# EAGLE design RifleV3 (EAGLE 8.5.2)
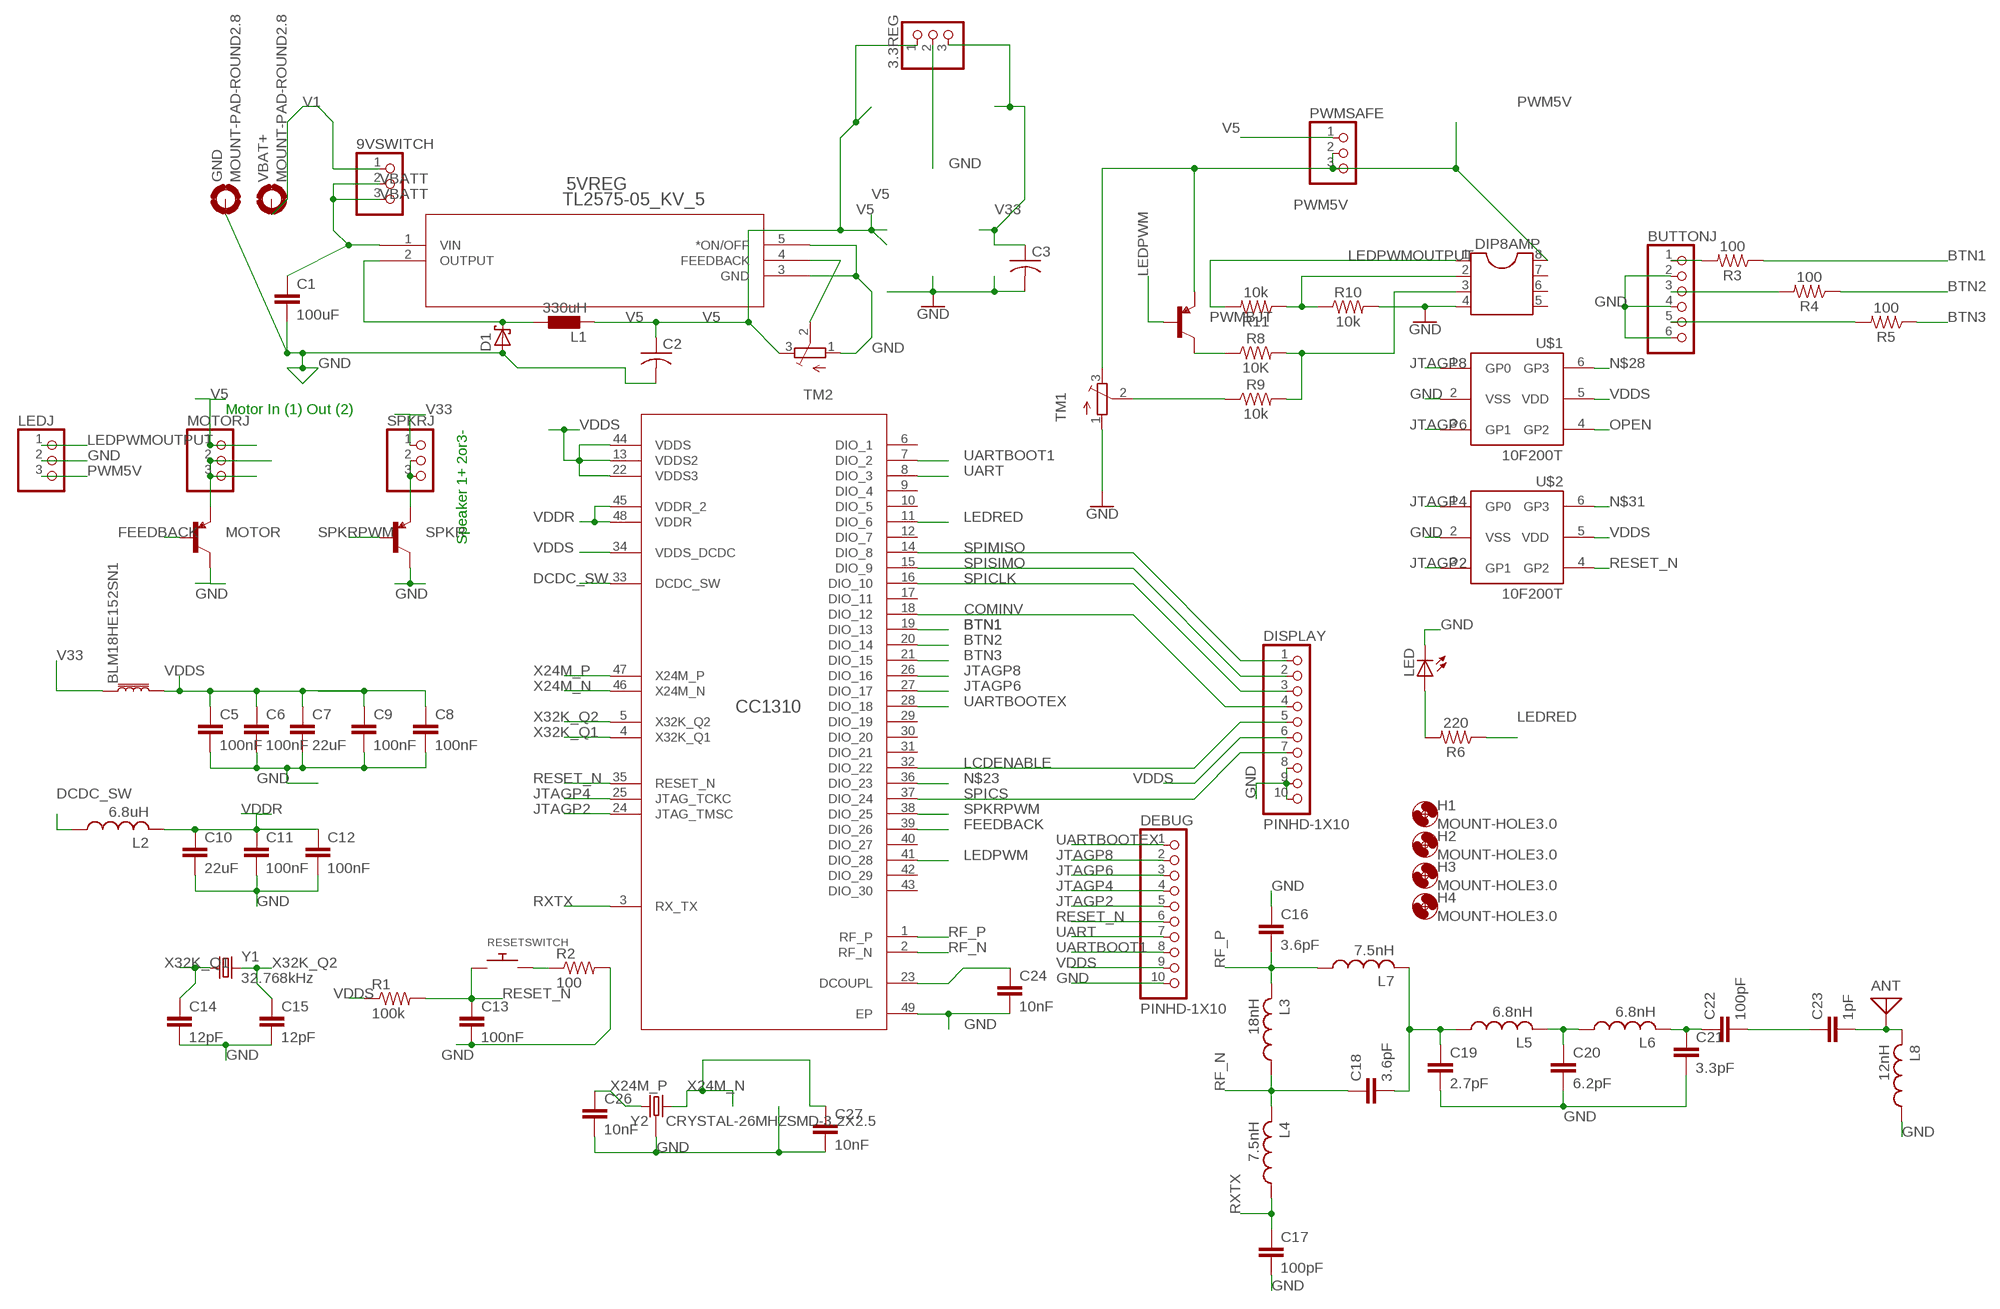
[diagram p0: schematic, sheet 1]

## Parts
3.3REG  PINHD-1X3CB  [1X03-CLEANBIG]
5VREG  TL2575-05_KV_5  [KV5]
9VSWITCH  PINHD-1X3  [1X03]
ANT  ANTENNA  [PAD-01]
BLM18HE152SN1  FERRITE_BEAD-0603  [0603]
BUTTONJ  PINHD-1X6  [1X06]
C1  100uF  10NF-PTH-10MM-10000V-1-%  [CAP-PTH-10MM]
C2  C-US025-024X044  [C025-024X044]
C3  C-US025-024X044  [C025-024X044]
C5  100nF  10NF-0603-50V-10%  [0603]
C6  100nF  10NF-0603-50V-10%  [0603]
C7  22uF  10NF-0603-50V-10%  [0603]
C8  100nF  10NF-0603-50V-10%  [0603]
C9  100nF  10NF-0603-50V-10%  [0603]
C10  22uF  10NF-0603-50V-10%  [0603]
C11  100nF  10NF-0603-50V-10%  [0603]
C12  100nF  10NF-0603-50V-10%  [0603]
C13  100nF  10NF-0603-50V-10%  [0603]
C14  12pF  10NF-0603-50V-10%  [0603]
C15  12pF  10NF-0603-50V-10%  [0603]
C16  3.6pF  10NF-0603-50V-10%  [0603]
C17  100pF  10NF-0603-50V-10%  [0603]
C18  3.6pF  10NF-0603-50V-10%  [0603]
C19  2.7pF  10NF-0603-50V-10%  [0603]
C20  6.2pF  10NF-0603-50V-10%  [0603]
C21  3.3pF  10NF-0603-50V-10%  [0603]
C22  100pF  10NF-0603-50V-10%  [0603]
C23  1pF  10NF-0603-50V-10%  [0603]
C24  10nF  10NF-0603-50V-10%  [0603]
C26  10nF  10NF-0603-50V-10%  [0603]
C27  10nF  10NF-0603-50V-10%  [0603]
CC1310  CC1310F128RGZR  [RGZ0048A]
D1  SCHOTTKY-DIODEDO41  [DO41-10]
DEBUG  PINHD-1X10  [1X10-BIG]
DIP8AMP  DIL8S  [SOCKET-08]
DISPLAY  PINHD-1X10  [1X10-BIG]
GND  MOUNT-PAD-ROUND2.8  [2,8-PAD]
H1  MOUNT-HOLE3.0  [3,0]
H2  MOUNT-HOLE3.0  [3,0]
H3  MOUNT-HOLE3.0  [3,0]
H4  MOUNT-HOLE3.0  [3,0]
L1  330uH  L0204/7  [0204/7]
L2  6.8uH  INDUCTOR_0603_M  [RESC0603_M]
L3  18nH  INDUCTOR_0603_M  [RESC0603_M]
L4  7.5nH  INDUCTOR_0603_M  [RESC0603_M]
L5  6.8nH  INDUCTOR_0603_M  [RESC0603_M]
L6  6.8nH  INDUCTOR_0603_M  [RESC0603_M]
L7  7.5nH  INDUCTOR_0603_M  [RESC0603_M]
L8  12nH  INDUCTOR_0603_M  [RESC0603_M]
LED  LEDCHIP-LED0805  [CHIP-LED0805]
LEDJ  PINHD-1X3  [1X03]
MOTOR  TRANSISTOR_PNPTO92  [TO-92]
MOTORJ  PINHD-1X3  [1X03]
PWMBJT  TRANSISTOR_PNPTO92  [TO-92]
PWMSAFE  PINHD-1X3  [1X03]
R1  100k  R-US_R0603  [R0603]
R2  100  R-US_R0603  [R0603]
R3  100  10MOHM-0603-1/10W-5%  [0603]
R4  100  10MOHM-0603-1/10W-5%  [0603]
R5  100  10MOHM-0603-1/10W-5%  [0603]
R6  220  10MOHM-0603-1/10W-5%  [0603]
R8  10K  10MOHM-0603-1/10W-5%  [0603]
R9  10k  10MOHM-0603-1/10W-5%  [0603]
R10  10k  10MOHM-0603-1/10W-5%  [0603]
R11  10k  10MOHM-0603-1/10W-5%  [0603]
RESETSWITCH  SWITCH_PUSHBUTTONSOFTTOUCHSMD_SJ  [PUSHBUTTON_SMD_SJ]
SPKR  TRANSISTOR_PNPTO92  [TO-92]
SPKRJ  PINHD-1X3  [1X03]
TM1  TRIMPOTTC33X  [TC33X]
TM2  TRIMPOTTC33X  [TC33X]
U$1  10F200T  [SOT23-6]
U$2  10F200T  [SOT23-6]
VBAT+  MOUNT-PAD-ROUND2.8  [2,8-PAD]
Y1  32.768kHz  FC-12M  [FC-12M]
Y2  CRYSTAL-26MHZSMD-3.2X2.5  [CRYSTAL-SMD-3.2X2.5MM]

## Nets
BTN1: CC1310.19(DIO_13) R3.1
BTN2: CC1310.20(DIO_14) R4.1
BTN3: CC1310.21(DIO_15) R5.1
COMINV: CC1310.18(DIO_12) DISPLAY.4
DCDC_SW: CC1310.33(DCDC_SW) L2.1
DCOUPL: C24.1 CC1310.23(DCOUPL)
FEEDBACK: CC1310.39(DIO_26) MOTOR.2(B)
GND: 3.3REG.2 5VREG.3(GND) 5VREG.5(*ON/OFF) BUTTONJ.2 BUTTONJ.4 BUTTONJ.6 C1.2 C2.2 C3.2 C5.2 C6.2 C7.2 C8.2 C9.2 C10.2 C11.2 C12.2 C13.2 C14.2 C15.2 C16.1 C17.2 C19.2 C20.2 C21.2 C24.2 C26.2 C27.2 CC1310.49(EP) D1.A DEBUG.10 DIP8AMP.4 DISPLAY.8 DISPLAY.9 DISPLAY.10 GND.B2,8(MOUNT) L8.1 LED.C LEDJ.2 MOTOR.3(C) R2.2 R10.2 SPKR.3(C) TM1.1(A) TM2.1(A) U$1.2(VSS) U$2.2(VSS) Y2.2 Y2.4
JTAGP2: CC1310.24(JTAG_TMSC) DEBUG.5 U$2.3(GP1)
JTAGP4: CC1310.25(JTAG_TCKC) DEBUG.4 U$2.1(GP0)
JTAGP6: CC1310.27(DIO_17) DEBUG.3 U$1.3(GP1)
JTAGP8: CC1310.26(DIO_16) DEBUG.2 U$1.1(GP0)
LCDENABLE: CC1310.32(DIO_22) DISPLAY.5
LEDPWM: CC1310.41(DIO_28) PWMBJT.2(B)
LEDPWMOUTPUT: DIP8AMP.1 LEDJ.1 R11.2
LEDRED: CC1310.11(DIO_6) R6.1
N$1: 5VREG.2(OUTPUT) D1.C L1.1
N$2: C22.2 C23.1
N$3: 5VREG.4(FEEDBACK) TM2.2(S)
N$4: MOTOR.1(E) MOTORJ.2 MOTORJ.3
N$5: C20.1 L5.2 L6.1
N$6: R2.1 RESETSWITCH.P$2
N$7: C18.2 C19.1 L5.1 L7.2
N$8: SPKR.1(E) SPKRJ.2 SPKRJ.3
N$9: ANT.1 C23.2 L8.2
N$10: R9.1 TM1.2(S)
N$11: PWMBJT.3(C) R8.1
N$12: BUTTONJ.1 R3.2
N$14: DIP8AMP.2 R10.1 R11.1
N$15: C21.1 C22.1 L6.2
N$16: DIP8AMP.3 R8.2 R9.2
N$17: BUTTONJ.3 R4.2
N$18: BUTTONJ.5 R5.2
N$22: LED.A R6.2
N$23: CC1310.36(DIO_23)
N$28: U$1.6(GP3)
N$31: U$2.6(GP3)
OPEN: U$1.4(GP2)
PWM5V: DIP8AMP.8 LEDJ.3 PWMBJT.1(E) PWMSAFE.2 PWMSAFE.3 TM1.3(E)
RESET_N: C13.1 CC1310.35(RESET_N) DEBUG.6 R1.2 RESETSWITCH.P$1 U$2.4(GP2)
RF_N: C18.1 CC1310.2(RF_N) L3.1 L4.2
RF_P: C16.2 CC1310.1(RF_P) L3.2 L7.1
RXTX: C17.1 CC1310.3(RX_TX) L4.1
SPICLK: CC1310.16(DIO_10) DISPLAY.3
SPICS: CC1310.37(DIO_24) DISPLAY.7
SPIMISO: CC1310.14(DIO_8) DISPLAY.1
SPISIMO: CC1310.15(DIO_9) DISPLAY.2
SPKRPWM: CC1310.38(DIO_25) SPKR.2(B)
UART: CC1310.8(DIO_3) DEBUG.7
UARTBOOT1: CC1310.7(DIO_2) DEBUG.8
UARTBOOTEX: CC1310.28(DIO_18) DEBUG.1
V1: 9VSWITCH.1 VBAT+.B2,8(MOUNT)
V5: 3.3REG.1 C2.1 L1.2 MOTORJ.1 PWMSAFE.1 TM2.3(E)
V33: 3.3REG.3 BLM18HE152SN1.1 C3.1 SPKRJ.1
VBATT: 5VREG.1(VIN) 9VSWITCH.2 9VSWITCH.3 C1.1
VDDR: C10.1 C11.1 C12.1 CC1310.45(VDDR_2) CC1310.48(VDDR) L2.2
VDDS: BLM18HE152SN1.2 C5.1 C6.1 C7.1 C8.1 C9.1 CC1310.13(VDDS2) CC1310.22(VDDS3) CC1310.34(VDDS_DCDC) CC1310.44(VDDS) DEBUG.9 DISPLAY.6 R1.1 U$1.5(VDD) U$2.5(VDD)
X24M_N: C27.1 CC1310.46(X24M_N) Y2.3
X24M_P: C26.1 CC1310.47(X24M_P) Y2.1
X32K_Q1: C14.1 CC1310.4(X32K_Q1) Y1.1
X32K_Q2: C15.1 CC1310.5(X32K_Q2) Y1.2
Unconnected: CC1310.6(DIO_1) CC1310.9(DIO_4) CC1310.10(DIO_5) CC1310.12(DIO_7) CC1310.17(DIO_11) CC1310.29(DIO_19) CC1310.30(DIO_20) CC1310.31(DIO_21) CC1310.40(DIO_27) CC1310.42(DIO_29) CC1310.43(DIO_30) DIP8AMP.5 DIP8AMP.6 DIP8AMP.7

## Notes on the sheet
- Motor In (1) Out (2)
- Speaker 1+ 2or3-

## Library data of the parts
3.3REG 9VSWITCH LEDJ MOTORJ PWMSAFE SPKRJ = adafruit:PINHD-1X3: PIN HEADER
5VREG = LM2575:TL2575-05_KV_5; DATASHEETURL: httpwww.ti.comlitgpnTL257505; FAMILY_NAME: STEPDOWN REGULATOR; GENERIC_PART_NUMBER: TL257505; INDUSTRY_STD_PKG_TYPE: TO220; MANUFACTURER: Texas Instruments; MANUFACTURER_PART_NUMBER: tl257505_kv_5; PACKAGE_DESIGNATOR: KV; PIN_COUNT: 5; VENDOR: Texas Instruments
ANT = discrete:ANTENNA: Antenna
BLM18HE152SN1 = SparkFun-Coils:FERRITE_BEAD: Ferrite Bead (blocks, cores, rings, chokes, etc.); PROD_ID: NDUC-07859; VALUE: 30Ω/1.8A
BUTTONJ = adafruit:PINHD-1X6: PIN HEADER
C1 = SparkFun-Capacitors:10NF: 0.01uF/10nF/10,000pF ceramic capacitors; PROD_ID: CAP-09321; VALUE: 10nF
C2 C3 = adafruit:C-US: CAPACITOR, American symbol
C5-C23 = SparkFun-Capacitors:10NF: 0.01uF/10nF/10,000pF ceramic capacitors; PROD_ID: CAP-00867; VALUE: 10nF
C24 C26 C27 = SparkFun-Capacitors:10NF: 0.01uF/10nF/10,000pF ceramic capacitors; PROD_ID: CAP-00867
CC1310 = CC1310RGZ:CC1310F128RGZR; ALTERNATEPARTNUMBER: CC1310F128RGZT; APPLICATION_BUILDNUMBER: *; COMPTYPE: IC; MANUFACTURER: Texas Instruments; MOUNTTYPE: SMT; PACKAGEREFERENCE: RGZ0048A; PARTNUMBER: CC1310F128RGZR; PIN_COUNT: 49; REFDES: RefDes; TYPE: TYPE; VALUE: Value
D1 = adafruit:SCHOTTKY-DIODE: Schottky Diode
DEBUG DISPLAY = adafruit:PINHD-1X10: Pin header 1x10 0.1" spacing With round pins
DIP8AMP = ic-package:DIL8: Dual In Line / Socket
GND VBAT+ = holes:MOUNT-PAD-ROUND: MOUNTING PAD, round
H1-H4 = holes:MOUNT-HOLE: MOUNTING HOLE with drill center marker
L1 = eagle-ltspice:L: INDUCTOR, European symbol; SPICEMODEL: NONE; SPICEPREFIX: L
L2-L8 = Nordic_nRF:INDUCTOR: Generic chip inductor
LED = adafruit:LED: LED
MOTOR PWMBJT SPKR = User-Submitted:TRANSISTOR_PNP: Generic PNP BJT Double check pinouts against datasheets- not all devices are the same! MMBT3906 - 40V 200mA SOT-23 (TRANS-08052) MMBT4403 - 40V 600mA SOT-23 (TRANS-09245)
R1 R2 = adafruit:R-US_: RESISTOR, American symbol
R3-R6 R8-R11 = SparkFun-Resistors:10MOHM: RES-09327; PROD_ID: RES-08283; VALUE: 10M
RESETSWITCH = adafruit:SWITCH_PUSHBUTTON: Buttons
TM1 TM2 = adafruit:TRIMPOT: SMT trimmer potentiometer part number TC33X http://www.ladyada.net/library/eagle
U$1 U$2 = adafruit:10F200T: PIC10F200/202/204/206 Ultra-small 8-bit PIC micros in SOT-23-6 and SOIC
Y1 = crystal:FC-12M: kHz RANGE CRYSTAL UNIT
Y2 = SparkFun-Clocks:CRYSTAL-26MHZ: 26MHz Crystal w/ Ground Pin Digikey Example Frequency: 26MHz Frequency Stability: &plusmn;9ppm Frequency Tolerance: &plusmn;10ppm Load Capacitance: 9pF SparkFun Products: SparkFun ESP32 Thing SparkFun ESP8266 Thing Dev Board; PROD_ID: XTAL-12454

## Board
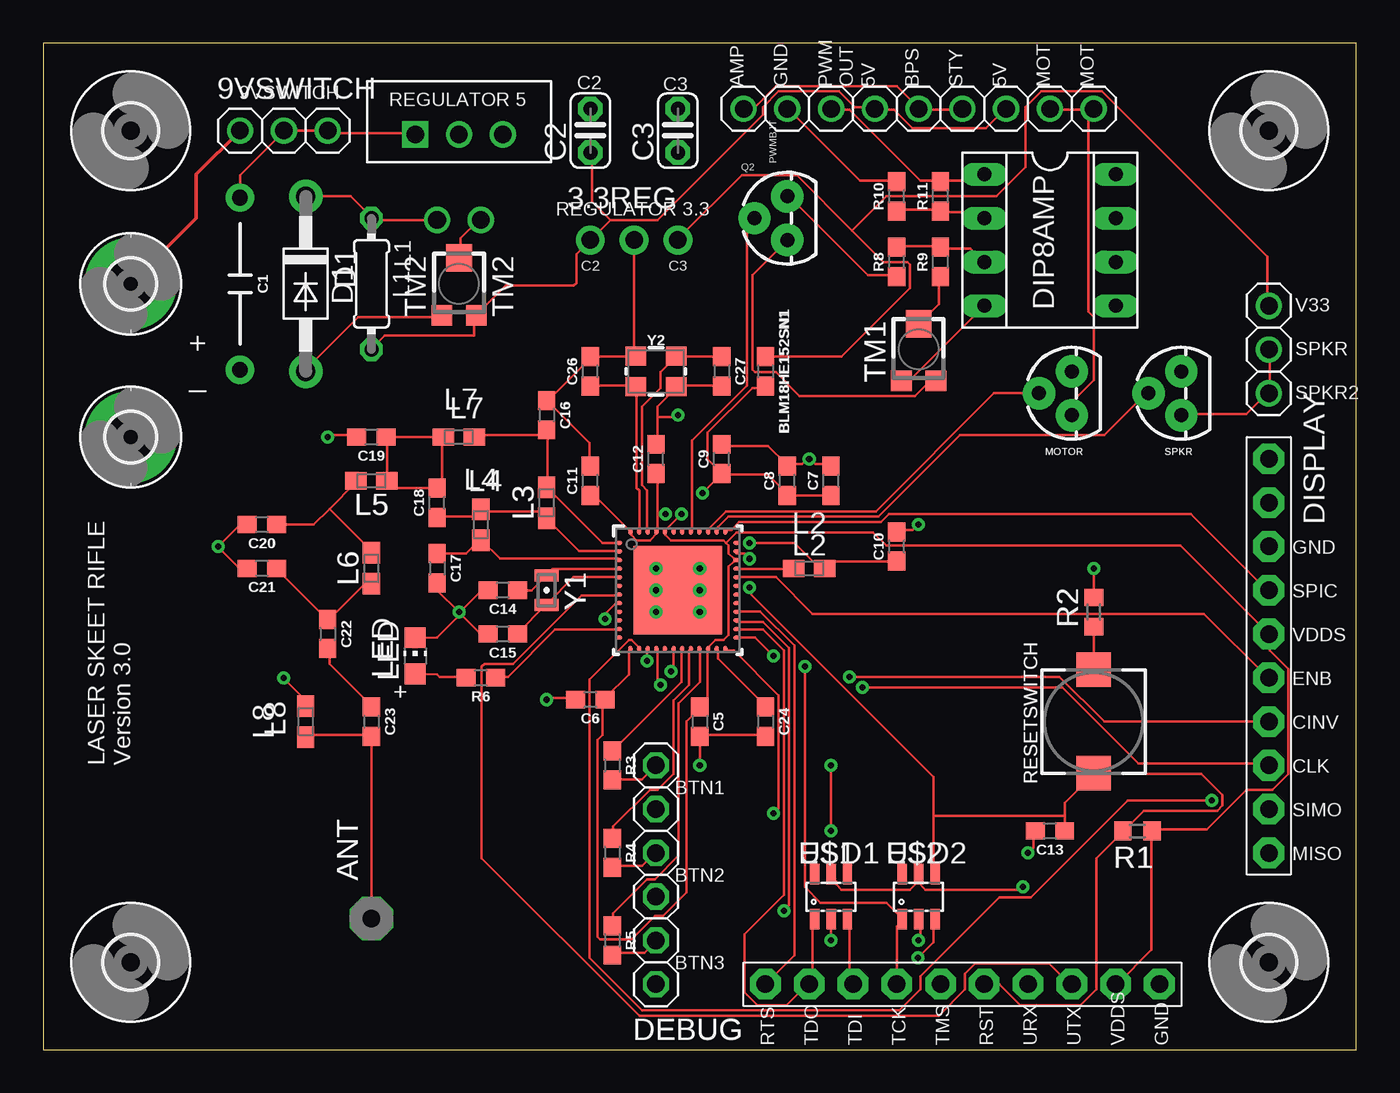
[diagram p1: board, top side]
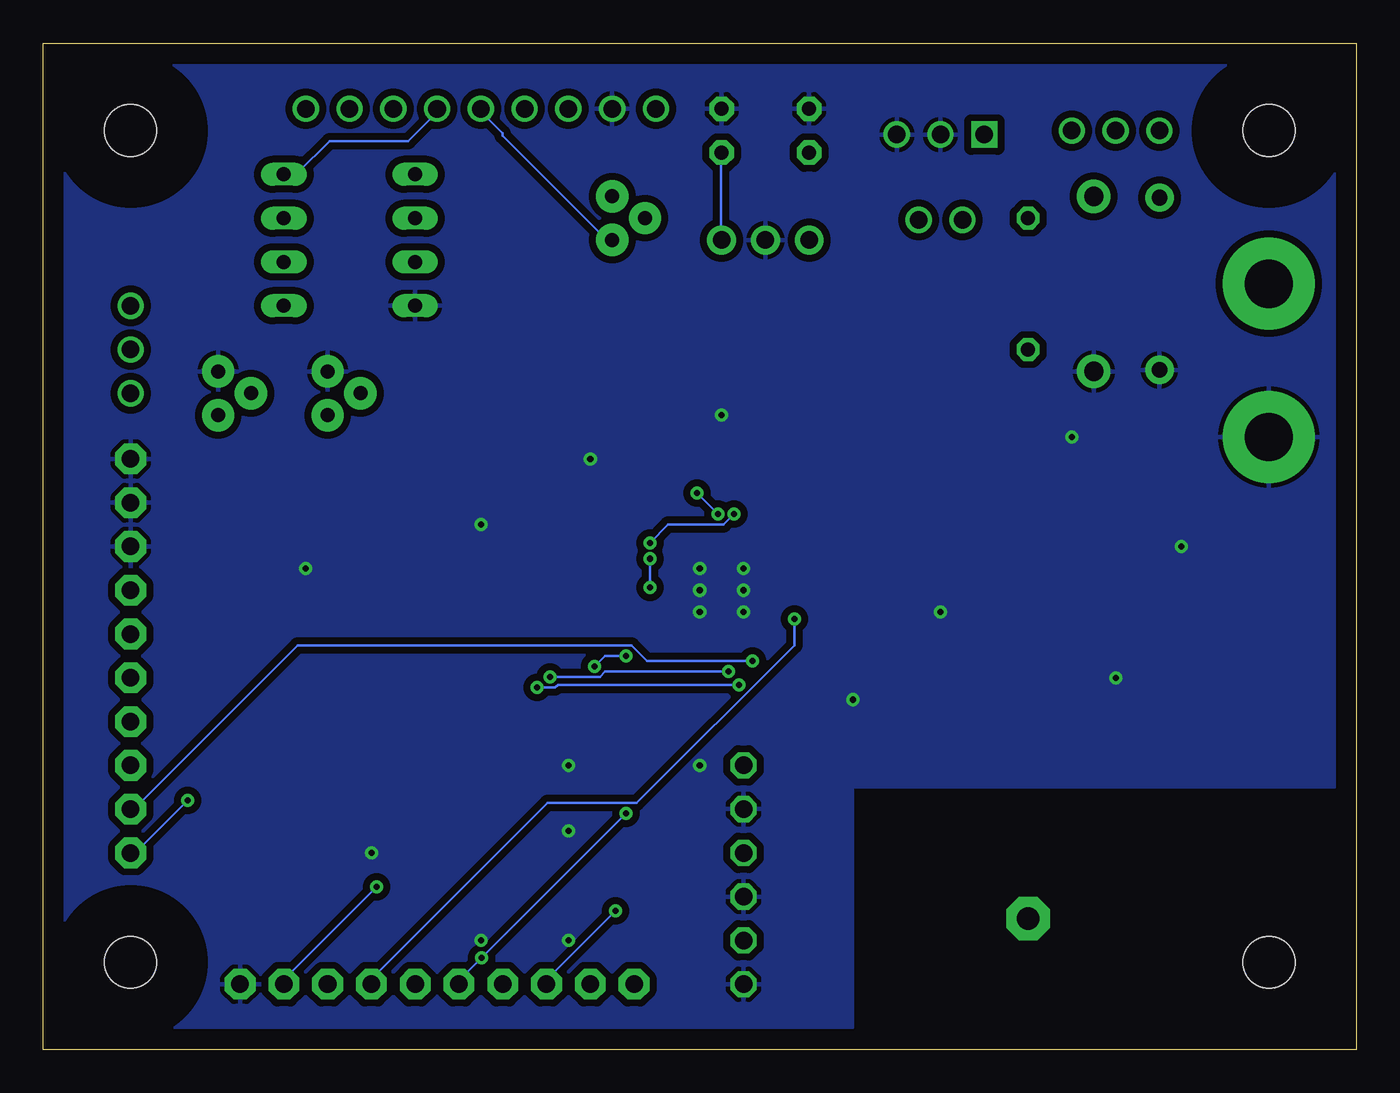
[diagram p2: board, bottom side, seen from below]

Size 76.2 x 58.42 mm. Coordinates in mm from the lower left corner, seen from the top.
Outline: 0,0 76.2,0 76.2,58.42 0,58.42 0,0
Copper layers (1*16): Top 0.035mm / dielectric 1.5mm / Bottom 0.035mm
Design rules "default": minimum track width 6mil, minimum drill 0.35mm, track to track 6mil, track to pad 6mil, pad to pad 6mil, via to via 6mil, smd to smd 6mil, copper to edge 40mil, drill to drill 6mil, minimum pad ring 10mil, minimum via ring 8mil, stop-mask expansion 4mil, vias tented up to drill 0mil, thermal gap 10mil

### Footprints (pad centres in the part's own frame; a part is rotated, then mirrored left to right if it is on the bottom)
1X03-CLEANBIG = drill 1.016 pad 1.676: 1 -2.54,0; 2 0,0; 3 2.54,0
KV5 = drill 1.016 pad 1.524 square: 1 -5.08,-1.499 | drill 1.016 pad 1.524: 2 -3.81,-6.452; 3 -2.54,-1.499; 4 -1.27,-6.452; 5 0,-1.499
1X03 = drill 1.016: 1 -2.54,0; 2 0,0; 3 2.54,0
PAD-01 = drill 1.321 pad 2.54 octagon: 1 0,0
0603 = smd 1.1 x 1: 1 -0.85,0; 2 0.85,0
1X06 = drill 1.016 octagon: 1 -6.35,0; 2 -3.81,0; 3 -1.27,0; 4 1.27,0; 5 3.81,0; 6 6.35,0
CAP-PTH-10MM = drill 0.9 pad 1.651: 1 -5,0; 2 5,0
C025-024X044 = drill 0.813 pad 1.422 octagon: 1 -1.27,0; 2 1.27,0
RGZ0048A = smd 0.36 x 0.24: 1 -3.4,2.75; 2 -3.4,2.25; 3 -3.4,1.75; 4 -3.4,1.25; 5 -3.4,0.75; 6 -3.4,0.25; 7 -3.4,-0.25; 8 -3.4,-0.75; 9 -3.4,-1.25; 10 -3.4,-1.75; 11 -3.4,-2.25; 12 -3.4,-2.75; 25 3.4,-2.75; 26 3.4,-2.25; 27 3.4,-1.75; 28 3.4,-1.25; 29 3.4,-0.75; 30 3.4,-0.25; 31 3.4,0.25; 32 3.4,0.75; 33 3.4,1.25; 34 3.4,1.75; 35 3.4,2.25; 36 3.4,2.75 | smd 0.24 x 0.36: 13 -2.75,-3.4; 14 -2.25,-3.4; 15 -1.75,-3.4; 16 -1.25,-3.4; 17 -0.75,-3.4; 18 -0.25,-3.4; 19 0.25,-3.4; 20 0.75,-3.4; 21 1.25,-3.4; 22 1.75,-3.4; 23 2.25,-3.4; 24 2.75,-3.4; 37 2.75,3.4; 38 2.25,3.4; 39 1.75,3.4; 40 1.25,3.4; 41 0.75,3.4; 42 0.25,3.4; 43 -0.25,3.4; 44 -0.75,3.4; 45 -1.25,3.4; 46 -1.75,3.4; 47 -2.25,3.4; 48 -2.75,3.4 | smd 5.15 x 5.15: 49 0,0 | smd 0.5 x 0.5: V -0.803,2.325
DO41-10 = drill 1.118 pad 1.93: A 5.08,0; C -5.08,0
1X10-BIG = drill 1.016 pad 1.778 octagon: 1 -11.43,0; 2 -8.89,0; 3 -6.35,0; 4 -3.81,0; 5 -1.27,0; 6 1.27,0; 7 3.81,0; 8 6.35,0; 9 8.89,0; 10 11.43,0
SOCKET-08 = drill 0.813 long: 1 -3.81,-3.81; 2 -1.27,-3.81; 3 1.27,-3.81; 4 3.81,-3.81; 5 3.81,3.81; 6 1.27,3.81; 7 -1.27,3.81; 8 -3.81,3.81
2,8-PAD = drill 2.8 pad 5.334: B2,8 0,0
3,0 = hole 3: 0,0
0204/7 = drill 0.813 octagon: 1 -3.81,0; 2 3.81,0
RESC0603_M = smd 1.25 x 1: 1 -0.9,0; 2 0.9,0
CHIP-LED0805 = smd 1.2 x 1.2: A 0,-1.05; C 0,1.05
TO-92 = drill 0.813 pad 1.88: 1 -1.27,0; 2 0,1.905; 3 1.27,0
R0603 = smd 1 x 1.1: 1 -0.85,0; 2 0.85,0
PUSHBUTTON_SMD_SJ = smd 2 x 2: P$1 3,0; P$2 -3,0
TC33X = smd 1.2 x 1.2: 1 -1,-1.825; 3 1,-1.825 | smd 1.5 x 1.6: 2 0,1.5
SOT23-6 = smd 0.55 x 1.2: 1 -0.95,-1.3; 2 0,-1.3; 3 0.95,-1.3; 4 0.95,1.3; 5 0,1.3; 6 -0.95,1.3
FC-12M = smd 0.7 x 1.4: 1 -0.85,0; 2 0.85,0
CRYSTAL-SMD-3.2X2.5MM = smd 1.2 x 1.1: 1 -1.175,-0.875; 2 1.175,-0.875; 3 1.175,0.875; 4 -1.175,0.875

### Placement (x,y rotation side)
3.3REG  34.29,46.99 0 top
5VREG  26.67,54.61 0 top
9VSWITCH  13.97,53.34 0 top
ANT  19.05,7.62 0 top
BLM18HE152SN1  41.91,39.37 270 top
BUTTONJ  35.56,10.16 270 top
C1  11.43,44.45 270 top
C2  31.75,53.34 90 top
C3  36.83,53.34 90 top
C5  38.1,19.05 270 top
C6  31.75,20.32 180 top
C7  45.72,33.02 90 top
C8  43.18,33.02 90 top
C9  39.37,34.29 90 top
C10  49.53,29.21 90 top
C11  31.75,33.02 90 top
C12  35.56,34.29 90 top
C13  58.42,12.7 180 top
C14  26.67,26.67 180 top
C15  26.67,24.13 180 top
C16  29.21,36.83 270 top
C17  22.86,27.94 270 top
C18  22.86,31.75 90 top
C19  19.05,35.56 180 top
C20  12.7,30.48 180 top
C21  12.7,27.94 180 top
C22  16.51,24.13 270 top
C23  19.05,19.05 270 top
C24  41.91,19.05 270 top
C26  31.75,39.37 90 top
C27  39.37,39.37 270 top
CC1310  36.83,26.67 0 top
D1  15.24,44.45 270 top
DEBUG  53.34,3.81 0 top
DIP8AMP  58.42,46.99 270 top
DISPLAY  71.12,22.86 90 top
GND  5.08,35.56 0 top
H1  71.12,5.08 0 top
H2  5.08,53.34 0 top
H3  71.12,53.34 0 top
H4  5.08,5.08 0 top
L1  19.05,44.45 270 top
L2  44.45,27.94 0 top
L3  29.21,31.75 90 top
L4  25.4,30.48 90 top
L5  19.05,33.02 180 top
L6  19.05,27.94 270 top
L7  24.13,35.56 180 top
L8  15.24,19.05 270 top
LED  21.59,22.86 0 top
LEDJ  43.18,54.61 180 top
MOTOR  59.69,38.1 90 top
MOTORJ  58.42,54.61 0 top
PWMBJT  43.18,48.26 90 top
PWMSAFE  50.8,54.61 0 top
R1  63.5,12.7 180 top
R2  60.96,25.4 90 top
R3  33.02,16.51 270 top
R4  33.02,11.43 270 top
R5  33.02,6.35 270 top
R6  25.4,21.59 180 top
R8  49.53,45.72 90 top
R9  52.07,45.72 90 top
R10  49.53,49.53 90 top
R11  52.07,49.53 90 top
RESETSWITCH  60.96,19.05 270 top
SPKR  66.04,38.1 90 top
SPKRJ  71.12,40.64 270 top
TM1  50.8,40.64 0 top
TM2  24.13,44.45 0 top
U$1  45.72,8.89 0 top
U$2  50.8,8.89 0 top
VBAT+  5.08,44.45 0 top
Y1  29.21,26.67 270 top
Y2  35.56,39.37 0 top

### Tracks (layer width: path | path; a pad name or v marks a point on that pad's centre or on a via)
BTN1
  Top 0.152: CC1310.19 37.03,23.16 37.03,21.34 33.07,17.37 R3.1
BTN2
  Top 0.152: CC1310.20 37.49,23.16 37.49,21.18 36.58,20.27 36.58,16 35.66,15.09 35.2,15.09 33.07,12.95 33.07,12.34 R4.1
BTN3
  Top 0.152: CC1310.21 38.1,23.16 38.1,21.34 36.88,20.12 36.88,11.28 35.51,9.91 35.05,9.91 33.07,7.92 33.07,7.32 R5.1
COMINV  (via drill 0.35)
  Top 0.152: v36.42,21.95 36.58,22.1 36.58,23.16 CC1310.18 | v46.79,21.64 58.98,21.64 61.57,19.05 DISPLAY.4
  Bottom 0.152: v36.42,21.95 43.59,21.95 43.89,21.64 v46.79,21.64
DCDC_SW
  Top 0.152: CC1310.33 40.23,27.89 43.43,27.89 L2.1
DCOUPL
  Top 0.152: CC1310.23 39.17,23.16 39.17,22.71 41.91,19.96 C24.1
FEEDBACK
  Top 0.152: MOTOR.2 55.17,38.1 48.31,31.24 39.62,31.24 38.56,30.18 CC1310.39
GND  (via drill 0.35)
  Top 0.152: 35.66,36.73 35.66,37.34 36.73,38.41 Y2.2 36.88,38.56 39.32,38.56 C27.2 | 35.66,36.73 35.66,35.2 C12.2 | C21.2 11.73,28.04 11.28,28.04 10.21,29.11 v10.16,29.21 11.43,30.48 C20.2 | C6.2 30.79,20.42 29.26,20.42 v29.21,20.32 | C19.2 18.14,35.66 16.61,35.66 v16.51,35.56 | v38.1,16.51 C5.2 38.1,18.29 41.91,18.29 C24.2 | 24.23,25.3 25.3,24.23 25.76,24.23 C15.2 | C17.2 22.86,26.67 v24.13,25.4 | C14.2 25.45,26.67 24.23,25.45 v24.13,25.4 | 29.26,37.64 31.7,35.2 31.7,33.98 C11.2 | v57.15,11.43 57.45,11.73 57.45,12.65 C13.2 | C10.2 49.53,30.18 50.44,30.18 50.75,30.48 v50.8,30.48 | v60.96,27.94 R2.2 | C7.2 45.72,33.98 44.81,33.98 44.5,34.29 v44.45,34.29 44.35,34.29 44.04,33.98 43.28,33.98 C8.2 43.13,33.98 42.06,35.05 39.47,35.05 C9.2 | R10.2 49.53,50.44 47.4,50.44 43.28,54.56 LEDJ.2 | v45.72,6.35 U$1.2 | U$2.2 50.9,7.47 50.9,6.4 v50.8,6.35 | 24.23,25.3 22.86,23.93 LED.C | 24.23,25.3 v24.13,25.4 | TM2.1 23.01,42.52 18.29,42.52 15.24,39.47 D1.A | DIP8AMP.4 50.29,38.86 49.84,38.86 TM1.1 | L8.1 15.24,20.27 14.02,21.49 v13.97,21.59 | v35.56,26.67 CC1310.49 | v45.72,12.7 v45.72,16.51 | 29.26,37.64 31.7,40.08 C26.2 31.85,40.23 34.29,40.23 Y2.4 34.29,40.39 3.3REG.2 | 29.26,37.64 C16.1 | 35.66,36.73 36.73,36.73 v36.83,36.83
  other vias: 35.56,27.94 38.1,27.94 35.56,25.4 38.1,25.4 38.1,26.67
  pour Bottom (isolate 0.406): 1.27,57.15 74.93,57.15 74.93,1.27 29.21,1.27 29.21,15.24 1.27,15.24
JTAGP2  (via drill 0.35)
  Top 0.152: v42.37,13.72 42.67,14.02 42.67,20.57 40.08,23.16 39.62,23.16 CC1310.24 | v50.75,5.33 51.66,6.25 51.66,7.47 U$2.3
  Bottom 0.152: v42.37,13.72 v50.75,5.33 51.97,4.12 51.97,3.81 DEBUG.5
JTAGP4  (via drill 0.35)
  Top 0.152: v42.37,22.86 41.3,23.93 CC1310.25 | v44.2,22.25 44.2,9.45 45.11,8.53 48.92,8.53 49.84,7.62 U$2.1 49.84,7.47 49.53,7.16 DEBUG.4
  Bottom 0.152: v42.37,22.86 43.59,22.86 v44.2,22.25
JTAGP6  (via drill 0.35)
  Top 0.152: v42.98,8.08 43.28,8.38 43.28,23.32 41.76,24.84 40.23,24.84 CC1310.27 | U$1.3 46.79,7.47 46.79,3.96 46.94,3.81 DEBUG.3
  Bottom 0.152: v42.98,8.08 46.94,4.12 46.94,3.81 DEBUG.3
JTAGP8
  Top 0.152: CC1310.26 40.23,24.38 41.76,24.38 42.98,23.16 42.98,8.99 40.69,6.71 40.69,3.35 41.45,2.59 43.13,2.59 44.35,3.81 DEBUG.2 44.5,3.81 44.65,3.96 44.65,7.47 U$1.1
LCDENABLE
  Top 0.152: CC1310.32 40.23,27.43 42.52,27.43 44.65,25.3 67.36,25.3 71.02,21.64 DISPLAY.5
LEDPWM
  Top 0.152: CC1310.41 37.64,30.18 37.64,35.36 40.84,38.56 40.84,47.85 41.15,48.16 PWMBJT.2
LEDPWMOUTPUT
  Top 0.152: DIP8AMP.1 54.25,50.44 52.12,50.44 R11.2 51.97,50.44 50.9,50.44 46.79,54.56 45.72,54.56 LEDJ.1
LEDRED
  Top 0.152: CC1310.11 33.38,24.38 29.72,24.38 26.98,21.64 26.36,21.64 R6.1
N$1
  Top 0.152: 5VREG.2 19.05,48.16 L1.1 19.05,48.31 17.83,49.53 D1.C
N$2
  Top 0.152: C22.2 16.61,23.16 16.61,22.4 19.05,19.96 C23.1
N$3
  Top 0.152: TM2.2 24.23,46.02 24.23,47.09 25.3,48.16 5VREG.4
N$4
  Top 0.152: 60.66,54.56 60.96,54.56 MOTORJ.3 60.66,54.56 | 60.66,54.56 58.52,54.56 MOTORJ.2 | 60.66,54.56 60.66,42.82 60.96,42.52 60.96,38.86 59.74,37.64 59.74,36.88 MOTOR.1
N$5
  Top 0.152: C20.1 15.7,30.48 16.61,31.39 | 16.61,31.39 18.14,32.92 L5.2 | 16.61,31.39 19.05,28.96 L6.1
N$6
  Top 0.152: RESETSWITCH.P$2 R2.1
N$7
  Top 0.152: 22.86,32.61 20.27,32.61 19.96,32.92 L5.1 19.96,33.07 19.96,35.51 C19.1 L7.2 23.16,35.51 23.16,32.92 22.86,32.61 | 22.86,32.61 C18.2
N$8
  Top 0.152: SPKRJ.2 71.17,40.54 71.17,38.1 SPKRJ.3 71.02,38.1 69.8,36.88 66.14,36.88 SPKR.1
N$9
  Top 0.152: L8.2 15.24,18.29 19.05,18.29 C23.2 ANT.1
N$10
  Top 0.152: R9.1 51.97,44.81 51.97,43.28 50.9,42.22 TM1.2
N$11
  Top 0.152: R8.1 49.53,44.96 47.85,44.96 43.28,49.53 PWMBJT.3
N$12
  Top 0.152: BUTTONJ.1 34.75,15.7 33.07,15.7 R3.2
N$14
  Top 0.152: R10.1 49.53,48.77 51.97,48.77 R11.1 52.12,48.62 54.25,48.62 DIP8AMP.2
N$15
  Top 0.152: C21.1 13.56,27.89 16.46,24.99 C22.1 16.61,24.99 18.59,26.98 19.05,26.98 L6.2
N$16
  Top 0.152: R8.2 49.53,46.63 51.97,46.63 R9.2 52.12,46.48 53.8,46.48 54.56,45.72 DIP8AMP.3
N$17
  Top 0.152: R4.2 33.07,10.67 34.75,10.67 35.51,11.43 BUTTONJ.3
N$18
  Top 0.152: R5.2 33.07,5.64 34.9,5.64 35.51,6.25 BUTTONJ.5
N$22
  Top 0.152: R6.2 24.54,21.64 23.01,21.64 22.86,21.79 LED.A
PWM5V
  Top 0.152: PWMBJT.1 41.15,44.96 41.15,39.47 41.3,39.32 42.52,39.32 43.89,37.95 50.6,37.95 51.36,38.71 51.66,38.71 TM1.3 | LEDJ.3 40.69,54.71 41.3,54.71 42.52,55.93 49.53,55.93 50.75,54.71 PWMSAFE.2 50.9,54.56 53.34,54.56 PWMSAFE.3
  Bottom 0.152: PWMSAFE.3 53.34,54.41 55.02,52.73 59.59,52.73 61.42,50.9 62.18,50.9 DIP8AMP.8 | PWMBJT.1 43.28,47.09 43.59,47.09 49.53,53.03 49.53,53.19 50.9,54.56 PWMSAFE.2
RESET_N  (via drill 0.35)
  Top 0.152: v41,28.5 40.69,28.8 40.23,28.8 CC1310.35 | v41,26.82 41,26.52 51.66,15.85 51.66,13.56 | 51.66,13.56 51.66,10.21 U$2.4 | 59.28,13.56 59.28,14.33 60.96,16 | 59.28,13.56 59.28,12.8 C13.1 | 60.96,16 67.21,16 68.43,14.78 68.43,14.17 68.12,13.87 63.86,13.87 62.79,12.8 R1.2 62.64,12.65 61.11,11.12 61.11,3.5 60.2,2.59 56.69,2.59 55.47,3.81 DEBUG.6 | 60.96,16 RESETSWITCH.P$1 | 59.28,13.56 51.66,13.56
  Bottom 0.152: v41,26.82 v41,28.5
RF_N
  Top 0.152: C18.1 22.86,30.94 24.99,30.94 25.3,31.24 L4.2 25.45,31.24 28.8,31.24 29.11,30.94 L3.1 29.26,30.79 31.09,28.96 33.38,28.96 CC1310.2
RF_P
  Top 0.152: CC1310.1 33.38,29.41 32.46,29.41 29.26,32.61 L3.2 29.26,32.77 29.26,35.66 | 29.26,35.66 29.26,35.97 C16.2 29.26,35.66 | 29.26,35.66 25.15,35.66 L7.1
RXTX
  Top 0.152: CC1310.3 33.38,28.5 26.52,28.5 25.45,29.57 L4.1 25.3,29.57 24.54,28.8 22.86,28.8 C17.1
SPICLK  (via drill 0.35)
  Top 0.152: v35.81,21.18 35.66,21.34 35.66,23.16 CC1310.16 | v47.55,21.03 59.13,21.03 63.55,16.61 71.02,16.61 DISPLAY.3
  Bottom 0.152: v35.81,21.18 46.33,21.18 46.48,21.03 v47.55,21.03
SPICS
  Top 0.152: CC1310.37 39.62,30.18 39.93,30.18 40.39,30.63 48.62,30.63 49.07,31.09 66.6,31.09 71.02,26.67 DISPLAY.7
SPIMISO  (via drill 0.35)
  Top 0.152: v67.82,14.48 62.94,14.48 57.3,8.84 55.47,8.84 50.9,4.27 50.9,3.5 49.68,2.29 34.75,2.29 31.7,5.33 31.7,21.49 33.98,23.77 34.14,23.77 34.59,23.32 CC1310.14
  Bottom 0.152: v67.82,14.48 70.87,11.43 DISPLAY.1
SPISIMO  (via drill 0.35)
  Top 0.152: v35.05,22.55 35.05,23.16 CC1310.15
  Bottom 0.152: v35.05,22.55 41.15,22.55 42.06,23.47 61.42,23.47 71.02,13.87 DISPLAY.2
SPKRPWM
  Top 0.152: CC1310.38 39.17,30.18 39.17,30.33 39.78,30.94 48.46,30.94 53.19,35.66 61.57,35.66 64.01,38.1 SPKR.2
UART  (via drill 0.35)
  Top 0.152: v32.61,24.99 32.61,25.3 33.22,25.91 33.38,25.91 CC1310.8
  Bottom 0.152: v32.61,24.99 32.61,23.47 41.76,14.33 46.94,14.33 57.15,4.12 DEBUG.7
UARTBOOT1
  Top 0.152: CC1310.7 33.38,26.36 31.24,26.36 27.28,22.4 25.6,22.4 25.45,22.25 25.45,11.12 34.59,1.98 51.97,1.98 53.49,3.5 53.49,4.42 54.1,5.03 58.37,5.03 59.59,3.81 DEBUG.8
UARTBOOTEX
  Top 0.152: DEBUG.1 43.59,5.49 43.59,23.47 41.6,25.45 40.23,25.45 CC1310.28
V1
  Top 0.203: VBAT+.B2,8 8.89,48.26 8.89,50.8 9VSWITCH.1
V5
  Top 0.152: MOTORJ.1 55.78,54.56 54.71,53.49 50.44,53.49 49.38,54.56 48.31,54.56 PWMSAFE.1 48.16,54.71 47.09,54.71 46.18,55.63 42.67,55.63 41.76,54.71 41.76,54.25 35.66,48.16 32.92,48.16 | L1.2 19.05,40.69 19.81,41.45 24.99,41.45 24.99,42.52 TM2.3 25.15,42.67 26.82,44.35 30.79,44.35 30.94,44.5 30.94,46.18 3.3REG.1 32.92,48.16 | 32.92,48.16 31.85,49.23 31.85,51.97 C2.1
V33
  Top 0.152: 46.94,47.55 43.74,50.75 40.54,50.75 36.88,47.09 3.3REG.3 | 46.94,47.55 48.77,45.72 50.14,45.72 50.29,45.57 50.29,44.2 46.33,40.23 41.91,40.23 BLM18HE152SN1.1 | 46.94,47.55 48.92,49.53 55.32,49.53 57,51.21 57,54.71 57.91,55.63 61.42,55.63 71.02,46.02 71.02,43.28 SPKRJ.1
  Bottom 0.152: C3.1 36.88,51.97 36.88,47.09 3.3REG.3
VBATT
  Top 0.152: 14.02,53.34 9VSWITCH.3 16.61,53.34 16.76,53.19 21.49,53.19 5VREG.1 | C1.1 11.43,50.75 14.02,53.34 | 14.02,53.34 9VSWITCH.2
VDDR  (via drill 0.35)
  Top 0.152: C10.1 49.53,28.35 45.72,28.35 45.41,28.04 L2.2 45.26,28.04 44.96,28.04 43.59,29.41 v41,29.41 | C11.1 31.85,32.31 33.98,30.18 CC1310.48 34.14,30.02 34.14,29.87 34.44,29.57 35.2,29.57 35.66,30.02 CC1310.45 35.66,30.18 35.66,31.09 | 35.66,31.09 35.66,33.38 C12.1 | 35.66,31.09 v36.12,31.09
  Bottom 0.152: v41,29.41 39.93,30.48 36.73,30.48 v36.12,31.09
VDDS  (via drill 0.35)
  Top 0.152: C7.1 45.72,32.16 43.28,32.16 C8.1 43.13,32.31 42.06,33.38 39.47,33.38 C9.1 | BLM18HE152SN1.2 41.91,38.41 41.15,38.41 38.56,35.81 38.56,34.29 39.32,33.53 C9.1 | CC1310.13 33.98,23.16 33.98,21.79 32.61,20.42 C6.1 32.46,20.27 32.46,18.29 32.16,17.98 32.16,6.55 32.31,6.4 34.14,6.4 35.51,7.77 35.97,7.77 37.34,9.14 37.34,19.05 38.1,19.81 C5.1 38.1,19.96 38.56,20.42 38.56,23.16 CC1310.22 38.56,23.32 39.01,23.77 39.47,23.77 39.78,24.08 39.78,28.04 40.08,28.35 CC1310.34 40.08,28.5 39.78,28.8 39.78,29.26 39.62,29.41 | 39.62,29.41 39.47,29.57 36.42,29.57 36.12,29.87 36.12,30.02 CC1310.44 36.12,30.18 v37.03,31.09 | v38.25,32.31 39.32,33.38 C9.1 | 50.75,9.75 50.29,9.3 46.33,9.3 46.02,9.6 46.02,9.75 45.72,10.06 U$1.5 | 50.75,9.75 50.75,10.06 U$2.5 50.75,9.75 | DEBUG.9 62.33,3.81 64.31,5.79 64.31,12.65 R1.1 64.47,12.8 67.51,12.8 69.8,15.09 71.32,15.09 72.24,16 72.24,22.1 71.17,23.16 71.17,24.08 DISPLAY.6 65.99,29.26 48.92,29.26 48.16,30.02 40.23,30.02 39.62,29.41 | 50.75,9.75 51.21,9.3 56.69,9.3 v56.84,9.45
  Bottom 0.152: v37.03,31.09 v38.25,32.31 | v56.84,9.45 62.18,4.12 62.18,3.81 DEBUG.9
X24M_N
  Top 0.152: CC1310.46 35.05,30.18 35.05,32.46 34.75,32.77 34.75,37.34 35.81,38.41 35.81,39.32 Y2.3 36.88,40.23 39.32,40.23 C27.1
X24M_P
  Top 0.152: CC1310.47 34.59,30.18 34.59,32.46 34.44,32.61 34.44,38.41 Y2.1 34.29,38.56 31.85,38.56 C26.1
X32K_Q1
  Top 0.152: CC1310.4 33.38,27.89 29.57,27.89 29.26,27.58 Y1.1 29.11,27.43 28.35,26.67 C14.1
X32K_Q2
  Top 0.152: CC1310.5 33.38,27.43 30.79,27.43 29.26,25.91 Y1.2 29.11,25.76 27.58,24.23 C15.1

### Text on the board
tNames: GND
_tNames: C2 | C3 | AMP | GND | PWM / OUT | 5V | BPS | STY | 5V | MOT | MOT | 9VSWITCH | REGULATOR 5 | Q2 | R10 | R11 | REGULATOR 3.3 | DIP8AMP | D1 | R8 | R9 | L1 | C2 | C3 | C1 | TM2 | V33 | Y2 | + / _ | SPKR | C26 | C27 | BLM18HE152SN1 | TM1 | SPKR2 | L7 | C16 | C19 | MOTOR | SPKR | C12 | C9 | C11 | C8 | C7 | L5 | C18 | L4 | L3 | C20 | DISPLAY | L2 | C10 | GND | C17 | Y1 | C21 | L6 | C14 | SPIC | R2 | C22 | VDDS | C15 | LED | R6 | ENB | C6 | RESETSWITCH | C23 | C5 | C24 | CINV | L8 | LASER SKEET RIFLE / Version 3.0 | R3 | CLK | BTN1 | SIMO | C13 | R1 | R4 | ESD1 | ESD2 | MISO | ANT | BTN2 | R5 | BTN3 | DEBUG | RTS | TDO | TDI | TCK | TMS | RST | URX | UTX | VDDS
200bmp: C:/Users/User/Desktop/laser.bmp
